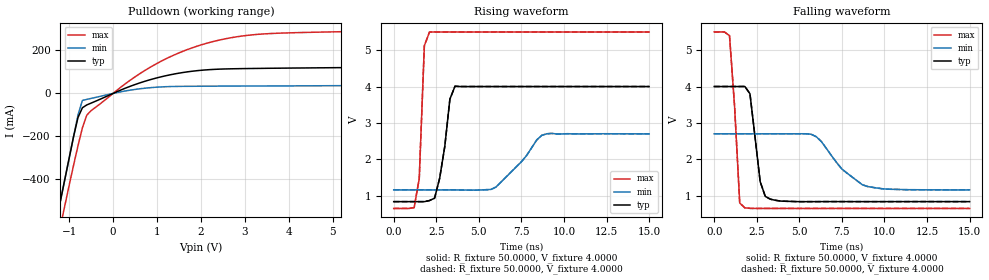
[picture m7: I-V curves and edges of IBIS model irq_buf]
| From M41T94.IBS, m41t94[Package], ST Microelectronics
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|   Model irq_buf
[Model]   irq_buf
Model_type   Open_drain
Polarity   Inverting
Vmeas =   1.5000V
Cref =1.000e-10F
Rref =   0.6450k
Vref =   1.7300V
C_comp   4.6000pF   3.1200pF   4.7300pF
[Temperature Range]   27.0000   85.0000   -40.0000
[Voltage Range]   4.0000V   2.7000V   5.5000V
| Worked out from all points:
|   slope of the pulldown table from 0 to 0.6 V, typ, clamps not added: 12.4 ohm
|   rising waveform, R_fixture 50.0000, V_fixture 4.0000: 20-80 % time 540ps typ, 1.7ns min, 239ps max; typ from 0.835 V to 4 V
|   rising waveform, R_fixture 50.0000, V_fixture 4.0000: 20-80 % time 540ps typ, 1.7ns min, 239ps max; typ from 0.835 V to 4 V
|   falling waveform, R_fixture 50.0000, V_fixture 4.0000: 20-80 % time 471ps typ, 1.78ns min, 374ps max; typ from 4 V to 0.835 V
|   falling waveform, R_fixture 50.0000, V_fixture 4.0000: 20-80 % time 471ps typ, 1.78ns min, 374ps max; typ from 4 V to 0.835 V
[Pulldown]
| voltage   I(typ)   I(min)   I(max)
-4V       -3.3A      -3.3A      -3.38A
-1.3V     -600mA     -600mA     -714mA
-1V       -300mA     -300mA     -426.8mA
-800mV    -112.2mA   -100mA     -243.5mA
-700mV    -66.89mA   -32.57mA   -160.4mA
-600mV    -53.66mA   -27.79mA   -101.3mA
-500mV    -45.06mA   -23.29mA   -79.97mA
500mV     41.34mA    18.54mA    77.23mA
1.3V      86.65mA    31.87mA    170.6mA
2.2V      110.7mA    33.62mA    237.4mA
3.5V      116.9mA    34.7mA     277.8mA
8V        131.5mA    41.4mA     305.1mA
[Ramp]
| variable   typ   min   max
dV/dt_r   2.3601/1.6721n   1.5627/1.8997n   3.2699/1.4981n
dV/dt_f   2.3604/0.2360n   1.5647/0.6007n   3.2700/0.2015n
R_load = 0.6450k
[Rising Waveform]
R_fixture = 50.0000
V_fixture = 4.0000
V_fixture_min = 2.7000
V_fixture_max = 5.5000
| time   V(typ)   V(min)   V(max)
0s        835.1mV    1.158V     647mV
1.2ns     835.1mV    1.158V     670.3mV
1.5ns     834.6mV    1.158V     1.47V
1.8ns     834.7mV    1.158V     5.121V
2.1ns     864.4mV    1.158V     5.497V
2.7ns     1.48V      1.158V     5.499V
3.6ns     4.009V     1.158V     5.5V
6ns       4V         1.234V     5.5V
9ns       4V         2.702V     5.5V
15ns      4V         2.698V     5.5V
[Rising Waveform]
R_fixture = 50.0000
V_fixture = 4.0000
V_fixture_min = 2.7000
V_fixture_max = 5.5000
| time   V(typ)   V(min)   V(max)
0s        835.1mV    1.158V     647mV
1.2ns     835.1mV    1.158V     670.3mV
1.5ns     834.6mV    1.158V     1.47V
1.8ns     834.7mV    1.158V     5.121V
2.1ns     864.4mV    1.158V     5.497V
2.7ns     1.48V      1.158V     5.499V
3.6ns     4.009V     1.158V     5.5V
6ns       4V         1.234V     5.5V
9ns       4V         2.702V     5.5V
15ns      4V         2.698V     5.5V
[Falling Waveform]
R_fixture = 50.0000
V_fixture = 4.0000
V_fixture_min = 2.7000
V_fixture_max = 5.5000
| time   V(typ)   V(min)   V(max)
0s        4V         2.7V       5.5V
900ps     4V         2.7V       5.398V
1.5ns     4V         2.7V       796.9mV
1.8ns     4.001V     2.7V       663.5mV
2.1ns     3.801V     2.7V       650mV
2.7ns     1.385V     2.7V       647.1mV
3.3ns     901.7mV    2.7V       646.5mV
6ns       834.8mV    2.619V     646.7mV
9ns       834.8mV    1.251V     646.6mV
15ns      834.9mV    1.159V     646.5mV
[Falling Waveform]
R_fixture = 50.0000
V_fixture = 4.0000
V_fixture_min = 2.7000
V_fixture_max = 5.5000
| time   V(typ)   V(min)   V(max)
0s        4V         2.7V       5.5V
900ps     4V         2.7V       5.398V
1.5ns     4V         2.7V       796.9mV
1.8ns     4.001V     2.7V       663.5mV
2.1ns     3.801V     2.7V       650mV
2.7ns     1.385V     2.7V       647.1mV
3.3ns     901.7mV    2.7V       646.5mV
6ns       834.8mV    2.619V     646.7mV
9ns       834.8mV    1.251V     646.6mV
15ns      834.9mV    1.159V     646.5mV
